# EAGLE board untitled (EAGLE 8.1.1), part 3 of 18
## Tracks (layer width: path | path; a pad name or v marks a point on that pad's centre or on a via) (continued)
S$2206 (continued)
  Bottom 0: 13.42,162.33 14.77,162.33
S$2207
  Bottom 0: 14.77,162.33 14.89,162.14
S$2208
  Bottom 0: 14.89,162.14 15.12,161.92
S$2209
  Bottom 0: 15.12,161.92 15.24,161.86
S$2210
  Bottom 0: 15.24,161.86 15.24,154.9
S$2211
  Bottom 0: 15.24,154.9 14.14,153.8
S$2212
  Bottom 0: 14.14,153.8 14.24,154.11
S$2213
  Bottom 0: 14.24,154.11 14.29,154.56
S$2214
  Bottom 0: 14.29,154.56 14.24,155.01
S$2215
  Bottom 0: 14.24,155.01 14.11,155.43
S$2216
  Bottom 0: 14.11,155.43 13.9,155.83
S$2217
  Bottom 0: 13.9,155.83 13.61,156.17
S$2218
  Bottom 0: 13.61,156.17 13.27,156.46
S$2219
  Bottom 0: 13.27,156.46 12.87,156.67
S$2220
  Bottom 0: 12.87,156.67 12.45,156.8
S$2221
  Bottom 0: 12.45,156.8 12,156.84
S$2222
  Bottom 0: 12,156.84 11.55,156.8
S$2223
  Bottom 0: 11.55,156.8 11.12,156.67
S$2224
  Bottom 0: 11.12,156.67 10.73,156.46
S$2225
  Bottom 0: 10.73,156.46 10.38,156.17
S$2226
  Bottom 0: 10.38,156.17 10.1,155.83
S$2227
  Bottom 0: 10.1,155.83 9.89,155.43
S$2228
  Bottom 0: 9.89,155.43 9.76,155.01
S$2229
  Bottom 0: 9.76,155.01 9.71,154.56
S$2230
  Bottom 0: 9.71,154.56 9.76,154.11
S$2231
  Bottom 0: 9.76,154.11 9.89,153.68
S$2232
  Bottom 0: 9.89,153.68 10.1,153.29
S$2233
  Bottom 0: 10.1,153.29 10.38,152.94
S$2234
  Bottom 0: 10.38,152.94 10.73,152.66
S$2235
  Bottom 0: 10.73,152.66 11.12,152.45
S$2236
  Bottom 0: 11.12,152.45 11.55,152.32
S$2237
  Bottom 0: 11.55,152.32 12,152.27
S$2238
  Bottom 0: 12,152.27 12.45,152.32
S$2239
  Bottom 0: 12.45,152.32 12.75,152.41
S$2240
  Bottom 0: 12.75,152.41 11.32,150.98
S$2241
  Bottom 0: 11.32,150.98 11.26,150.92
S$2242
  Bottom 0: 11.26,150.92 11.22,150.84
S$2243
  Bottom 0: 11.22,150.84 11.18,150.76
S$2244
  Bottom 0: 11.18,150.76 11.16,150.67
S$2245
  Bottom 0: 11.16,150.67 11.16,150.58
S$2246
  Bottom 0: 11.16,150.58 11.16,139.25
S$2247
  Bottom 0: 11.16,139.25 11.16,139.18
S$2248
  Bottom 0: 11.16,139.18 0.88,128.9
S$2249
  Bottom 0: 0.88,128.9 0.82,128.83
S$2250
  Bottom 0: 0.82,128.83 0.78,128.75
S$2251
  Bottom 0: 0.78,128.75 0.74,128.67
S$2252
  Bottom 0: 0.74,128.67 0.72,128.59
S$2253
  Bottom 0: 0.72,128.59 0.71,128.49
S$2254
  Bottom 0: 0.71,128.49 0.71,104.63
S$2255
  Bottom 0: 0.71,104.63 0.59,104.57
S$2256
  Bottom 0: 0.59,104.57 0.36,104.34
S$2257
  Bottom 0: 0.36,104.34 0.19,104.07
S$2258
  Bottom 0: 0.19,104.07 0.1,103.75
S$2259
  Bottom 0: 0.1,103.75 0.1,103.43
S$2260
  Bottom 0: 0.1,103.43 0.19,103.11
S$2261
  Bottom 0: 0.19,103.11 0.36,102.84
S$2262
  Bottom 0: 0.36,102.84 0.59,102.62
S$2263
  Bottom 0: 0.59,102.62 0.88,102.47
S$2264
  Bottom 0: 0.88,102.47 1.2,102.4
S$2265
  Bottom 0: 1.2,102.4 1.53,102.42
S$2266
  Bottom 0: 1.53,102.42 1.83,102.53
S$2267
  Bottom 0: 1.83,102.53 2.1,102.72
S$2268
  Bottom 0: 2.1,102.72 2.3,102.97
S$2269
  Bottom 0: 2.3,102.97 2.43,103.27
S$2270
  Bottom 0: 2.43,103.27 2.48,103.59
S$2271
  Bottom 0: 2.48,103.59 2.43,103.91
S$2272
  Bottom 0: 2.43,103.91 2.3,104.21
S$2273
  Bottom 0: 2.3,104.21 2.1,104.47
S$2274
  Bottom 0: 2.1,104.47 1.85,104.64
S$2275
  Bottom 0: 1.85,104.64 1.85,128.26
S$2276
  Bottom 0: 1.85,128.26 12.11,138.53
S$2277
  Bottom 0: 12.11,138.53 16.02,138.53
S$2278
  Bottom 0: 16.02,138.53 19.37,135.17
S$2279
  Bottom 0: 19.37,135.17 19.37,133.7
S$2280
  Bottom 0: 19.37,133.7 19.21,133.92
S$2281
  Bottom 0: 19.21,133.92 18.94,134.15
S$2282
  Bottom 0: 18.94,134.15 18.62,134.3
S$2283
  Bottom 0: 18.62,134.3 18.27,134.36
S$2284
  Bottom 0: 18.27,134.36 17.93,134.34
S$2285
  Bottom 0: 17.93,134.34 17.59,134.23
S$2286
  Bottom 0: 17.59,134.23 17.3,134.05
S$2287
  Bottom 0: 17.3,134.05 17.06,133.79
S$2288
  Bottom 0: 17.06,133.79 16.89,133.48
S$2289
  Bottom 0: 16.89,133.48 16.8,133.14
S$2290
  Bottom 0: 16.8,133.14 16.8,132.79
S$2291
  Bottom 0: 16.8,132.79 16.89,132.46
S$2292
  Bottom 0: 16.89,132.46 16.95,132.35
S$2293
  Bottom 0: 16.95,132.35 9.29,124.7
S$2294
  Bottom 0: 9.29,124.7 9.21,124.59
S$2295
  Bottom 0: 9.21,124.59 9.19,124.53
S$2296
  Bottom 0: 9.19,124.53 9.17,124.46
S$2297
  Bottom 0: 9.17,124.46 9.16,124.39
S$2298
  Bottom 0: 9.16,124.39 9.16,103.63
S$2299
  Bottom 0: 9.16,103.63 7.46,103.63
S$2300
  Bottom 0: 7.46,103.63 7.38,103.62
S$2301
  Bottom 0: 7.38,103.62 7.32,103.58
S$2302
  Bottom 0: 7.32,103.58 7.26,103.53
S$2303
  Bottom 0: 7.26,103.53 7.22,103.45
S$2304
  Bottom 0: 7.22,103.45 7.21,103.38
S$2305
  Bottom 0: 7.21,103.38 7.21,102.93
S$2306
  Bottom 0: 7.21,102.93 7.08,102.93
S$2307
  Bottom 0: 7.08,102.93 6.86,102.87
S$2308
  Bottom 0: 6.86,102.87 6.7,102.71
S$2309
  Bottom 0: 6.7,102.71 6.64,102.49
S$2310
  Bottom 0: 6.64,102.49 6.64,101.96
S$2311
  Bottom 0: 6.64,101.96 1.75,97.06
S$2312
  Bottom 0: 1.75,97.06 1.53,97.14
S$2313
  Bottom 0: 1.53,97.14 1.2,97.16
S$2314
  Bottom 0: 1.2,97.16 0.88,97.09
S$2315
  Bottom 0: 0.88,97.09 0.59,96.95
S$2316
  Bottom 0: 0.59,96.95 0.36,96.72
S$2317
  Bottom 0: 0.36,96.72 0.19,96.45
S$2318
  Bottom 0: 0.19,96.45 0.1,96.13
S$2319
  Bottom 0: 0.1,96.13 0.1,95.81
S$2320
  Bottom 0: 0.1,95.81 0.19,95.49
S$2321
  Bottom 0: 0.19,95.49 0.36,95.22
S$2322
  Bottom 0: 0.36,95.22 0.59,95
S$2323
  Bottom 0: 0.59,95 0.88,94.85
S$2324
  Bottom 0: 0.88,94.85 1.2,94.78
S$2325
  Bottom 0: 1.2,94.78 1.53,94.8
S$2326
  Bottom 0: 1.53,94.8 1.83,94.91
S$2327
  Bottom 0: 1.83,94.91 2.1,95.1
S$2328
  Bottom 0: 2.1,95.1 2.3,95.35
S$2329
  Bottom 0: 2.3,95.35 2.43,95.65
S$2330
  Bottom 0: 2.43,95.65 2.48,95.97
S$2331
  Bottom 0: 2.48,95.97 2.43,96.29
S$2332
  Bottom 0: 2.43,96.29 2.37,96.43
S$2333
  Bottom 0: 2.37,96.43 7.33,101.39
S$2334
  Bottom 0: 7.33,101.39 7.38,101.36
S$2335
  Bottom 0: 7.38,101.36 7.46,101.35
S$2336
  Bottom 0: 7.46,101.35 9.16,101.35
S$2337
  Bottom 0: 9.16,101.35 9.16,100.84
S$2338
  Bottom 0: 9.16,100.84 9.17,100.77
S$2339
  Bottom 0: 9.17,100.77 9.19,100.7
S$2340
  Bottom 0: 9.19,100.7 9.21,100.64
S$2341
  Bottom 0: 9.21,100.64 9.25,100.58
S$2342
  Bottom 0: 9.25,100.58 9.29,100.52
S$2343
  Bottom 0: 9.29,100.52 10.21,99.61
S$2344
  Bottom 0: 10.21,99.61 10.07,99.65
S$2345
  Bottom 0: 10.07,99.65 9.62,99.69
S$2346
  Bottom 0: 9.62,99.69 9.17,99.65
S$2347
  Bottom 0: 9.17,99.65 8.75,99.52
S$2348
  Bottom 0: 8.75,99.52 8.35,99.31
S$2349
  Bottom 0: 8.35,99.31 8,99.02
S$2350
  Bottom 0: 8,99.02 7.72,98.68
S$2351
  Bottom 0: 7.72,98.68 7.51,98.28
S$2352
  Bottom 0: 7.51,98.28 7.38,97.86
S$2353
  Bottom 0: 7.38,97.86 7.33,97.41
S$2354
  Bottom 0: 7.33,97.41 7.38,96.96
S$2355
  Bottom 0: 7.38,96.96 7.51,96.53
S$2356
  Bottom 0: 7.51,96.53 7.72,96.14
S$2357
  Bottom 0: 7.72,96.14 8,95.79
S$2358
  Bottom 0: 8,95.79 8.35,95.51
S$2359
  Bottom 0: 8.35,95.51 8.75,95.3
S$2360
  Bottom 0: 8.75,95.3 9.17,95.17
S$2361
  Bottom 0: 9.17,95.17 9.62,95.12
S$2362
  Bottom 0: 9.62,95.12 10.07,95.17
S$2363
  Bottom 0: 10.07,95.17 10.49,95.3
S$2364
  Bottom 0: 10.49,95.3 10.89,95.51
S$2365
  Bottom 0: 10.89,95.51 11.24,95.79
S$2366
  Bottom 0: 11.24,95.79 11.52,96.14
S$2367
  Bottom 0: 11.52,96.14 11.73,96.53
S$2368
  Bottom 0: 11.73,96.53 11.86,96.96
S$2369
  Bottom 0: 11.86,96.96 11.91,97.41
S$2370
  Bottom 0: 11.91,97.41 11.86,97.86
S$2371
  Bottom 0: 11.86,97.86 11.82,97.99
S$2372
  Bottom 0: 11.82,97.99 13.56,96.25
S$2373
  Bottom 0: 13.56,96.25 13.52,96.26
S$2374
  Bottom 0: 13.52,96.26 13.16,96.24
S$2375
  Bottom 0: 13.16,96.24 12.84,96.13
S$2376
  Bottom 0: 12.84,96.13 12.54,95.95
S$2377
  Bottom 0: 12.54,95.95 12.3,95.69
S$2378
  Bottom 0: 12.3,95.69 12.13,95.38
S$2379
  Bottom 0: 12.13,95.38 12.04,95.04
S$2380
  Bottom 0: 12.04,95.04 12.04,94.7
S$2381
  Bottom 0: 12.04,94.7 12.13,94.36
S$2382
  Bottom 0: 12.13,94.36 12.3,94.05
S$2383
  Bottom 0: 12.3,94.05 12.54,93.79
S$2384
  Bottom 0: 12.54,93.79 12.84,93.6
S$2385
  Bottom 0: 12.84,93.6 13.16,93.5
S$2386
  Bottom 0: 13.16,93.5 13.52,93.48
S$2387
  Bottom 0: 13.52,93.48 13.86,93.54
S$2388
  Bottom 0: 13.86,93.54 14.18,93.69
S$2389
  Bottom 0: 14.18,93.69 14.45,93.91
S$2390
  Bottom 0: 14.45,93.91 14.65,94.2
S$2391
  Bottom 0: 14.65,94.2 14.78,94.52
S$2392
  Bottom 0: 14.78,94.52 14.83,94.87
S$2393
  Bottom 0: 14.83,94.87 14.81,95.01
S$2394
  Bottom 0: 14.81,95.01 15.72,94.09
S$2395
  Bottom 0: 15.72,94.09 15.72,92.14
S$2396
  Bottom 0: 15.72,92.14 15.73,92.07
S$2397
  Bottom 0: 15.73,92.07 15.74,92
S$2398
  Bottom 0: 15.74,92 15.77,91.94
S$2399
  Bottom 0: 15.77,91.94 15.81,91.88
S$2400
  Bottom 0: 15.81,91.88 15.85,91.83
S$2401
  Bottom 0: 15.85,91.83 16.39,91.28
S$2402
  Bottom 0: 16.39,91.28 8.75,91.28
S$2403
  Bottom 0: 8.75,91.28 8.32,91.71
S$2404
  Bottom 0: 8.32,91.71 8.43,91.98
S$2405
  Bottom 0: 8.43,91.98 8.48,92.33
S$2406
  Bottom 0: 8.48,92.33 8.43,92.67
S$2407
  Bottom 0: 8.43,92.67 8.3,93
S$2408
  Bottom 0: 8.3,93 8.1,93.28
S$2409
  Bottom 0: 8.1,93.28 7.83,93.51
S$2410
  Bottom 0: 7.83,93.51 7.51,93.66
S$2411
  Bottom 0: 7.51,93.66 7.17,93.72
S$2412
  Bottom 0: 7.17,93.72 6.82,93.7
S$2413
  Bottom 0: 6.82,93.7 6.49,93.59
S$2414
  Bottom 0: 6.49,93.59 6.19,93.41
S$2415
  Bottom 0: 6.19,93.41 5.95,93.15
S$2416
  Bottom 0: 5.95,93.15 5.78,92.84
S$2417
  Bottom 0: 5.78,92.84 5.7,92.5
S$2418
  Bottom 0: 5.7,92.5 5.7,92.16
S$2419
  Bottom 0: 5.7,92.16 5.78,91.82
S$2420
  Bottom 0: 5.78,91.82 5.95,91.51
S$2421
  Bottom 0: 5.95,91.51 6.19,91.25
S$2422
  Bottom 0: 6.19,91.25 6.49,91.06
S$2423
  Bottom 0: 6.49,91.06 6.82,90.96
S$2424
  Bottom 0: 6.82,90.96 7.17,90.94
S$2425
  Bottom 0: 7.17,90.94 7.51,91
S$2426
  Bottom 0: 7.51,91 7.7,91.08
S$2427
  Bottom 0: 7.7,91.08 8.25,90.53
S$2428
  Bottom 0: 8.25,90.53 8.3,90.48
S$2429
  Bottom 0: 8.3,90.48 8.36,90.45
S$2430
  Bottom 0: 8.36,90.45 8.43,90.42
S$2431
  Bottom 0: 8.43,90.42 8.49,90.4
S$2432
  Bottom 0: 8.49,90.4 8.56,90.4
S$2433
  Bottom 0: 275.48,90.92 275.78,90.98
S$2434
  Bottom 0: 275.78,90.98 275.89,90.94
S$2435
  Bottom 0: 275.89,90.94 276.24,90.92
S$2436
  Bottom 0: 276.24,90.92 276.59,90.98
S$2437
  Bottom 0: 276.59,90.98 276.9,91.14
S$2438
  Bottom 0: 276.9,91.14 277.17,91.36
S$2439
  Bottom 0: 277.17,91.36 277.38,91.64
S$2440
  Bottom 0: 277.38,91.64 277.5,91.97
S$2441
  Bottom 0: 277.5,91.97 277.55,92.31
S$2442
  Bottom 0: 277.55,92.31 277.5,92.66
S$2443
  Bottom 0: 277.5,92.66 277.38,92.98
S$2444
  Bottom 0: 277.38,92.98 277.17,93.27
S$2445
  Bottom 0: 277.17,93.27 276.9,93.49
S$2446
  Bottom 0: 276.9,93.49 276.59,93.64
S$2447
  Bottom 0: 276.59,93.64 276.24,93.71
S$2448
  Bottom 0: 276.24,93.71 275.89,93.69
S$2449
  Bottom 0: 275.89,93.69 275.78,93.65
S$2450
  Bottom 0: 275.78,93.65 275.48,93.71
S$2451
  Bottom 0: 275.48,93.71 275.13,93.69
S$2452
  Bottom 0: 275.13,93.69 274.8,93.58
S$2453
  Bottom 0: 274.8,93.58 274.5,93.39
S$2454
  Bottom 0: 274.5,93.39 274.26,93.14
S$2455
  Bottom 0: 274.26,93.14 274.09,92.83
S$2456
  Bottom 0: 274.09,92.83 274.07,92.76
S$2457
  Bottom 0: 274.07,92.76 270.91,92.76
S$2458
  Bottom 0: 270.91,92.76 270.16,93.5
S$2459
  Bottom 0: 270.16,93.5 270.18,93.53
S$2460
  Bottom 0: 270.18,93.53 270.22,93.83
S$2461
  Bottom 0: 270.22,93.83 270.18,94.13
S$2462
  Bottom 0: 270.18,94.13 270.04,94.4
S$2463
  Bottom 0: 270.04,94.4 269.84,94.62
S$2464
  Bottom 0: 269.84,94.62 269.57,94.77
S$2465
  Bottom 0: 269.57,94.77 269.28,94.84
S$2466
  Bottom 0: 269.28,94.84 268.98,94.82
S$2467
  Bottom 0: 268.98,94.82 268.69,94.71
S$2468
  Bottom 0: 268.69,94.71 268.46,94.52
S$2469
  Bottom 0: 268.46,94.52 268.29,94.27
S$2470
  Bottom 0: 268.29,94.27 268.2,93.98
S$2471
  Bottom 0: 268.2,93.98 268.2,93.67
S$2472
  Bottom 0: 268.2,93.67 268.29,93.39
S$2473
  Bottom 0: 268.29,93.39 268.46,93.14
S$2474
  Bottom 0: 268.46,93.14 268.69,92.95
S$2475
  Bottom 0: 268.69,92.95 268.98,92.84
S$2476
  Bottom 0: 268.98,92.84 269.28,92.82
S$2477
  Bottom 0: 269.28,92.82 269.53,92.87
S$2478
  Bottom 0: 269.53,92.87 270.4,92
S$2479
  Bottom 0: 270.4,92 270.46,91.96
S$2480
  Bottom 0: 270.46,91.96 270.52,91.92
S$2481
  Bottom 0: 270.52,91.92 270.58,91.89
S$2482
  Bottom 0: 270.58,91.89 270.65,91.88
S$2483
  Bottom 0: 270.65,91.88 270.72,91.87
S$2484
  Bottom 0: 270.72,91.87 274.07,91.87
S$2485
  Bottom 0: 274.07,91.87 274.09,91.8
S$2486
  Bottom 0: 274.09,91.8 274.26,91.49
S$2487
  Bottom 0: 274.26,91.49 274.5,91.24
S$2488
  Bottom 0: 274.5,91.24 274.8,91.05
S$2489
  Bottom 0: 274.8,91.05 275.13,90.94
S$2490
  Bottom 0: 275.13,90.94 275.48,90.92
S$2491
  Bottom 0: 197.67,90.94 198.01,91
S$2492
  Bottom 0: 198.01,91 198.33,91.15
S$2493
  Bottom 0: 198.33,91.15 198.6,91.37
S$2494
  Bottom 0: 198.6,91.37 198.81,91.66
S$2495
  Bottom 0: 198.81,91.66 198.93,91.98
S$2496
  Bottom 0: 198.93,91.98 198.98,92.33
S$2497
  Bottom 0: 198.98,92.33 198.93,92.67
S$2498
  Bottom 0: 198.93,92.67 198.81,93
S$2499
  Bottom 0: 198.81,93 198.6,93.28
S$2500
  Bottom 0: 198.6,93.28 198.33,93.51
S$2501
  Bottom 0: 198.33,93.51 198.01,93.66
S$2502
  Bottom 0: 198.01,93.66 197.67,93.72
S$2503
  Bottom 0: 197.67,93.72 197.31,93.7
S$2504
  Bottom 0: 197.31,93.7 196.99,93.59
S$2505
  Bottom 0: 196.99,93.59 196.96,93.57
S$2506
  Bottom 0: 196.96,93.57 193.44,97.09
S$2507
  Bottom 0: 193.44,97.09 193.44,104.83
S$2508
  Bottom 0: 193.44,104.83 193.63,104.94
S$2509
  Bottom 0: 193.63,104.94 193.83,105.16
S$2510
  Bottom 0: 193.83,105.16 193.97,105.43
S$2511
  Bottom 0: 193.97,105.43 194.01,105.73
S$2512
  Bottom 0: 194.01,105.73 193.97,106.03
S$2513
  Bottom 0: 193.97,106.03 193.83,106.3
S$2514
  Bottom 0: 193.83,106.3 193.63,106.52
S$2515
  Bottom 0: 193.63,106.52 193.37,106.67
S$2516
  Bottom 0: 193.37,106.67 193.07,106.74
S$2517
  Bottom 0: 193.07,106.74 192.77,106.72
S$2518
  Bottom 0: 192.77,106.72 192.49,106.61
S$2519
  Bottom 0: 192.49,106.61 192.25,106.42
S$2520
  Bottom 0: 192.25,106.42 192.08,106.17
S$2521
  Bottom 0: 192.08,106.17 191.99,105.88
S$2522
  Bottom 0: 191.99,105.88 191.99,105.58
S$2523
  Bottom 0: 191.99,105.58 192.08,105.29
S$2524
  Bottom 0: 192.08,105.29 192.25,105.04
S$2525
  Bottom 0: 192.25,105.04 192.49,104.85
S$2526
  Bottom 0: 192.49,104.85 192.55,104.83
S$2527
  Bottom 0: 192.55,104.83 192.55,96.91
S$2528
  Bottom 0: 192.55,96.91 192.56,96.84
S$2529
  Bottom 0: 192.56,96.84 192.57,96.77
S$2530
  Bottom 0: 192.57,96.77 192.6,96.71
S$2531
  Bottom 0: 192.6,96.71 192.64,96.65
S$2532
  Bottom 0: 192.64,96.65 192.68,96.6
S$2533
  Bottom 0: 192.68,96.6 196.34,92.94
S$2534
  Bottom 0: 196.34,92.94 196.28,92.84
S$2535
  Bottom 0: 196.28,92.84 196.19,92.5
S$2536
  Bottom 0: 196.19,92.5 196.19,92.16
S$2537
  Bottom 0: 196.19,92.16 196.28,91.82
S$2538
  Bottom 0: 196.28,91.82 196.45,91.51
S$2539
  Bottom 0: 196.45,91.51 196.69,91.25
S$2540
  Bottom 0: 196.69,91.25 196.99,91.06
S$2541
  Bottom 0: 196.99,91.06 197.31,90.96
S$2542
  Bottom 0: 197.31,90.96 197.67,90.94
S$2543
  Bottom 0: 126.23,90.94 126.58,91
S$2544
  Bottom 0: 126.58,91 126.89,91.15
S$2545
  Bottom 0: 126.89,91.15 127.16,91.37
S$2546
  Bottom 0: 127.16,91.37 127.37,91.66
S$2547
  Bottom 0: 127.37,91.66 127.5,91.98
S$2548
  Bottom 0: 127.5,91.98 127.54,92.33
S$2549
  Bottom 0: 127.54,92.33 127.5,92.67
S$2550
  Bottom 0: 127.5,92.67 127.37,93
S$2551
  Bottom 0: 127.37,93 127.16,93.28
S$2552
  Bottom 0: 127.16,93.28 126.89,93.51
S$2553
  Bottom 0: 126.89,93.51 126.58,93.66
S$2554
  Bottom 0: 126.58,93.66 126.23,93.72
S$2555
  Bottom 0: 126.23,93.72 125.88,93.7
S$2556
  Bottom 0: 125.88,93.7 125.55,93.59
S$2557
  Bottom 0: 125.55,93.59 125.53,93.58
S$2558
  Bottom 0: 125.53,93.58 121.99,97.11
S$2559
  Bottom 0: 121.99,97.11 121.99,104.83
S$2560
  Bottom 0: 121.99,104.83 122.18,104.94
S$2561
  Bottom 0: 122.18,104.94 122.39,105.16
S$2562
  Bottom 0: 122.39,105.16 122.52,105.44
S$2563
  Bottom 0: 122.52,105.44 122.56,105.73
S$2564
  Bottom 0: 122.56,105.73 122.52,106.03
S$2565
  Bottom 0: 122.52,106.03 122.39,106.31
S$2566
  Bottom 0: 122.39,106.31 122.18,106.53
S$2567
  Bottom 0: 122.18,106.53 121.92,106.68
S$2568
  Bottom 0: 121.92,106.68 121.62,106.75
S$2569
  Bottom 0: 121.62,106.75 121.32,106.73
S$2570
  Bottom 0: 121.32,106.73 121.04,106.61
S$2571
  Bottom 0: 121.04,106.61 120.8,106.43
S$2572
  Bottom 0: 120.8,106.43 120.64,106.18
S$2573
  Bottom 0: 120.64,106.18 120.54,105.89
S$2574
  Bottom 0: 120.54,105.89 120.54,105.58
S$2575
  Bottom 0: 120.54,105.58 120.64,105.29
S$2576
  Bottom 0: 120.64,105.29 120.8,105.04
S$2577
  Bottom 0: 120.8,105.04 121.04,104.86
S$2578
  Bottom 0: 121.04,104.86 121.11,104.83
S$2579
  Bottom 0: 121.11,104.83 121.11,96.93
S$2580
  Bottom 0: 121.11,96.93 121.11,96.86
S$2581
  Bottom 0: 121.11,96.86 121.13,96.79
S$2582
  Bottom 0: 121.13,96.79 121.15,96.73
S$2583
  Bottom 0: 121.15,96.73 121.19,96.67
S$2584
  Bottom 0: 121.19,96.67 121.23,96.61
S$2585
  Bottom 0: 121.23,96.61 124.9,92.94
S$2586
  Bottom 0: 124.9,92.94 124.85,92.84
S$2587
  Bottom 0: 124.85,92.84 124.76,92.5
S$2588
  Bottom 0: 124.76,92.5 124.76,92.16
S$2589
  Bottom 0: 124.76,92.16 124.85,91.82
S$2590
  Bottom 0: 124.85,91.82 125.02,91.51
S$2591
  Bottom 0: 125.02,91.51 125.26,91.25
S$2592
  Bottom 0: 125.26,91.25 125.55,91.06
S$2593
  Bottom 0: 125.55,91.06 125.88,90.96
S$2594
  Bottom 0: 125.88,90.96 126.23,90.94
S$2595
  Bottom 0: 54.79,90.94 55.14,91
S$2596
  Bottom 0: 55.14,91 55.45,91.15
S$2597
  Bottom 0: 55.45,91.15 55.72,91.37
S$2598
  Bottom 0: 55.72,91.37 55.93,91.66
S$2599
  Bottom 0: 55.93,91.66 56.06,91.98
S$2600
  Bottom 0: 56.06,91.98 56.1,92.33
S$2601
  Bottom 0: 56.1,92.33 56.06,92.67
S$2602
  Bottom 0: 56.06,92.67 55.93,93
S$2603
  Bottom 0: 55.93,93 55.72,93.28
S$2604
  Bottom 0: 55.72,93.28 55.45,93.51
S$2605
  Bottom 0: 55.45,93.51 55.14,93.66
S$2606
  Bottom 0: 55.14,93.66 54.79,93.72
S$2607
  Bottom 0: 54.79,93.72 54.44,93.7
S$2608
  Bottom 0: 54.44,93.7 54.11,93.59
S$2609
  Bottom 0: 54.11,93.59 54.09,93.58
S$2610
  Bottom 0: 54.09,93.58 53.52,94.14
S$2611
  Bottom 0: 53.52,94.14 53.47,94.18
S$2612
  Bottom 0: 53.47,94.18 53.41,94.22
S$2613
  Bottom 0: 53.41,94.22 53.34,94.25
S$2614
  Bottom 0: 53.34,94.25 53.28,94.26
S$2615
  Bottom 0: 53.28,94.26 53.21,94.27
S$2616
  Bottom 0: 53.21,94.27 49.82,94.27
S$2617
  Bottom 0: 49.82,94.27 49.75,94.4
S$2618
  Bottom 0: 49.75,94.4 49.55,94.62
S$2619
  Bottom 0: 49.55,94.62 49.28,94.77
S$2620
  Bottom 0: 49.28,94.77 48.99,94.84
S$2621
  Bottom 0: 48.99,94.84 48.68,94.82
S$2622
  Bottom 0: 48.68,94.82 48.41,94.71
S$2623
  Bottom 0: 48.41,94.71 48.17,94.52
S$2624
  Bottom 0: 48.17,94.52 48,94.27
S$2625
  Bottom 0: 48,94.27 47.91,93.98
S$2626
  Bottom 0: 47.91,93.98 47.91,93.67
S$2627
  Bottom 0: 47.91,93.67 48,93.39
S$2628
  Bottom 0: 48,93.39 48.17,93.14
S$2629
  Bottom 0: 48.17,93.14 48.41,92.95
S$2630
  Bottom 0: 48.41,92.95 48.68,92.84
S$2631
  Bottom 0: 48.68,92.84 48.99,92.82
S$2632
  Bottom 0: 48.99,92.82 49.28,92.88
S$2633
  Bottom 0: 49.28,92.88 49.55,93.03
S$2634
  Bottom 0: 49.55,93.03 49.75,93.25
S$2635
  Bottom 0: 49.75,93.25 49.82,93.39
S$2636
  Bottom 0: 49.82,93.39 53.02,93.39
S$2637
  Bottom 0: 53.02,93.39 53.46,92.94
S$2638
  Bottom 0: 53.46,92.94 53.41,92.84
S$2639
  Bottom 0: 53.41,92.84 53.32,92.5
S$2640
  Bottom 0: 53.32,92.5 53.32,92.16
S$2641
  Bottom 0: 53.32,92.16 53.41,91.82
S$2642
  Bottom 0: 53.41,91.82 53.58,91.51
S$2643
  Bottom 0: 53.58,91.51 53.82,91.25
S$2644
  Bottom 0: 53.82,91.25 54.11,91.06
S$2645
  Bottom 0: 54.11,91.06 54.44,90.96
S$2646
  Bottom 0: 54.44,90.96 54.79,90.94
S$2647
  Bottom 0: 316.02,95.11 316.4,95.15
S$2648
  Bottom 0: 316.4,95.15 316.78,95.11
S$2649
  Bottom 0: 316.78,95.11 317.23,95.16
S$2650
  Bottom 0: 317.23,95.16 317.65,95.29
S$2651
  Bottom 0: 317.65,95.29 318.05,95.5
S$2652
  Bottom 0: 318.05,95.5 318.4,95.78
S$2653
  Bottom 0: 318.4,95.78 318.68,96.13
S$2654
  Bottom 0: 318.68,96.13 318.9,96.53
S$2655
  Bottom 0: 318.9,96.53 319.02,96.95
S$2656
  Bottom 0: 319.02,96.95 319.07,97.4
S$2657
  Bottom 0: 319.07,97.4 319.02,97.85
S$2658
  Bottom 0: 319.02,97.85 318.9,98.27
S$2659
  Bottom 0: 318.9,98.27 318.68,98.67
S$2660
  Bottom 0: 318.68,98.67 318.4,99.01
S$2661
  Bottom 0: 318.4,99.01 318.05,99.3
S$2662
  Bottom 0: 318.05,99.3 317.65,99.51
S$2663
  Bottom 0: 317.65,99.51 317.23,99.64
S$2664
  Bottom 0: 317.23,99.64 316.78,99.69
S$2665
  Bottom 0: 316.78,99.69 316.4,99.64
S$2666
  Bottom 0: 316.4,99.64 316.02,99.69
S$2667
  Bottom 0: 316.02,99.69 315.57,99.64
S$2668
  Bottom 0: 315.57,99.64 315.15,99.51
S$2669
  Bottom 0: 315.15,99.51 314.75,99.3
S$2670
  Bottom 0: 314.75,99.3 314.41,99.01
S$2671
  Bottom 0: 314.41,99.01 314.12,98.67
S$2672
  Bottom 0: 314.12,98.67 313.91,98.27
S$2673
  Bottom 0: 313.91,98.27 313.78,97.85
S$2674
  Bottom 0: 313.78,97.85 313.74,97.4
S$2675
  Bottom 0: 313.74,97.4 313.78,96.95
S$2676
  Bottom 0: 313.78,96.95 313.91,96.53
S$2677
  Bottom 0: 313.91,96.53 314.12,96.13
S$2678
  Bottom 0: 314.12,96.13 314.41,95.78
S$2679
  Bottom 0: 314.41,95.78 314.75,95.5
S$2680
  Bottom 0: 314.75,95.5 315.15,95.29
S$2681
  Bottom 0: 315.15,95.29 315.57,95.16
S$2682
  Bottom 0: 315.57,95.16 316.02,95.11
S$2683
  Bottom 0: 200.12,95.12 200.57,95.17
S$2684
  Bottom 0: 200.57,95.17 201,95.3
S$2685
  Bottom 0: 201,95.3 201.39,95.51
S$2686
  Bottom 0: 201.39,95.51 201.74,95.79
S$2687
  Bottom 0: 201.74,95.79 202.02,96.14
S$2688
  Bottom 0: 202.02,96.14 202.24,96.53
S$2689
  Bottom 0: 202.24,96.53 202.36,96.96
S$2690
  Bottom 0: 202.36,96.96 202.41,97.41
S$2691
  Bottom 0: 202.41,97.41 202.36,97.86
S$2692
  Bottom 0: 202.36,97.86 202.24,98.28
S$2693
  Bottom 0: 202.24,98.28 202.02,98.68
S$2694
  Bottom 0: 202.02,98.68 201.74,99.02
S$2695
  Bottom 0: 201.74,99.02 201.39,99.31
S$2696
  Bottom 0: 201.39,99.31 201,99.52
S$2697
  Bottom 0: 201,99.52 200.57,99.65
S$2698
  Bottom 0: 200.57,99.65 200.12,99.69
S$2699
  Bottom 0: 200.12,99.69 199.67,99.65
S$2700
  Bottom 0: 199.67,99.65 199.25,99.52
S$2701
  Bottom 0: 199.25,99.52 198.85,99.31
S$2702
  Bottom 0: 198.85,99.31 198.51,99.02
S$2703
  Bottom 0: 198.51,99.02 198.22,98.68
S$2704
  Bottom 0: 198.22,98.68 198.01,98.28
S$2705
  Bottom 0: 198.01,98.28 197.88,97.86
S$2706
  Bottom 0: 197.88,97.86 197.84,97.41
S$2707
  Bottom 0: 197.84,97.41 197.88,96.96
S$2708
  Bottom 0: 197.88,96.96 198.01,96.53
S$2709
  Bottom 0: 198.01,96.53 198.22,96.14
S$2710
  Bottom 0: 198.22,96.14 198.51,95.79
S$2711
  Bottom 0: 198.51,95.79 198.85,95.51
S$2712
  Bottom 0: 198.85,95.51 199.25,95.3
S$2713
  Bottom 0: 199.25,95.3 199.67,95.17
S$2714
  Bottom 0: 199.67,95.17 200.12,95.12
S$2715
  Bottom 0: 128.69,95.12 129.13,95.17
S$2716
  Bottom 0: 129.13,95.17 129.56,95.3
S$2717
  Bottom 0: 129.56,95.3 129.96,95.51
S$2718
  Bottom 0: 129.96,95.51 130.3,95.79
S$2719
  Bottom 0: 130.3,95.79 130.59,96.14
S$2720
  Bottom 0: 130.59,96.14 130.8,96.53
S$2721
  Bottom 0: 130.8,96.53 130.93,96.96
S$2722
  Bottom 0: 130.93,96.96 130.97,97.41
S$2723
  Bottom 0: 130.97,97.41 130.93,97.86
S$2724
  Bottom 0: 130.93,97.86 130.8,98.28
S$2725
  Bottom 0: 130.8,98.28 130.59,98.68
S$2726
  Bottom 0: 130.59,98.68 130.3,99.02
S$2727
  Bottom 0: 130.3,99.02 129.96,99.31
S$2728
  Bottom 0: 129.96,99.31 129.56,99.52
S$2729
  Bottom 0: 129.56,99.52 129.13,99.65
S$2730
  Bottom 0: 129.13,99.65 128.69,99.69
S$2731
  Bottom 0: 128.69,99.69 128.24,99.65
S$2732
  Bottom 0: 128.24,99.65 127.81,99.52
S$2733
  Bottom 0: 127.81,99.52 127.42,99.31
S$2734
  Bottom 0: 127.42,99.31 127.07,99.02
S$2735
  Bottom 0: 127.07,99.02 126.79,98.68
S$2736
  Bottom 0: 126.79,98.68 126.57,98.28
S$2737
  Bottom 0: 126.57,98.28 126.45,97.86
S$2738
  Bottom 0: 126.45,97.86 126.4,97.41
S$2739
  Bottom 0: 126.4,97.41 126.45,96.96
S$2740
  Bottom 0: 126.45,96.96 126.57,96.53
S$2741
  Bottom 0: 126.57,96.53 126.79,96.14
S$2742
  Bottom 0: 126.79,96.14 127.07,95.79
S$2743
  Bottom 0: 127.07,95.79 127.42,95.51
S$2744
  Bottom 0: 127.42,95.51 127.81,95.3
S$2745
  Bottom 0: 127.81,95.3 128.24,95.17
S$2746
  Bottom 0: 128.24,95.17 128.69,95.12
S$2747
  Bottom 0: 306.29,95.89 306.81,95.89
S$2748
  Bottom 0: 306.81,95.89 307.31,95.98
S$2749
  Bottom 0: 307.31,95.98 307.81,96.14
S$2750
  Bottom 0: 307.81,96.14 308.26,96.39
S$2751
  Bottom 0: 308.26,96.39 308.67,96.71
S$2752
  Bottom 0: 308.67,96.71 309.02,97.09
S$2753
  Bottom 0: 309.02,97.09 309.31,97.52
S$2754
  Bottom 0: 309.31,97.52 309.51,98
S$2755
  Bottom 0: 309.51,98 309.64,98.5
S$2756
  Bottom 0: 309.64,98.5 309.68,99.01
S$2757
  Bottom 0: 309.68,99.01 309.64,99.53
S$2758
  Bottom 0: 309.64,99.53 309.51,100.03
S$2759
  Bottom 0: 309.51,100.03 309.31,100.51
S$2760
  Bottom 0: 309.31,100.51 309.02,100.94
S$2761
  Bottom 0: 309.02,100.94 308.67,101.32
S$2762
  Bottom 0: 308.67,101.32 308.26,101.64
S$2763
  Bottom 0: 308.26,101.64 307.81,101.88
S$2764
  Bottom 0: 307.81,101.88 307.31,102.05
S$2765
  Bottom 0: 307.31,102.05 306.81,102.14
S$2766
  Bottom 0: 306.81,102.14 306.29,102.14
S$2767
  Bottom 0: 306.29,102.14 305.78,102.05
S$2768
  Bottom 0: 305.78,102.05 305.29,101.88
S$2769
  Bottom 0: 305.29,101.88 304.84,101.64
S$2770
  Bottom 0: 304.84,101.64 304.42,101.32
S$2771
  Bottom 0: 304.42,101.32 304.07,100.94
S$2772
  Bottom 0: 304.07,100.94 303.79,100.51
S$2773
  Bottom 0: 303.79,100.51 303.58,100.03
S$2774
  Bottom 0: 303.58,100.03 303.45,99.53
S$2775
  Bottom 0: 303.45,99.53 303.41,99.01
S$2776
  Bottom 0: 303.41,99.01 303.45,98.5
S$2777
  Bottom 0: 303.45,98.5 303.58,98
S$2778
  Bottom 0: 303.58,98 303.79,97.52
S$2779
  Bottom 0: 303.79,97.52 304.07,97.09
S$2780
  Bottom 0: 304.07,97.09 304.42,96.71
S$2781
  Bottom 0: 304.42,96.71 304.84,96.39
S$2782
  Bottom 0: 304.84,96.39 305.29,96.14
S$2783
  Bottom 0: 305.29,96.14 305.78,95.98
S$2784
  Bottom 0: 305.78,95.98 306.29,95.89
S$2785
  Bottom 0: 169.95,96.17 170.28,96.19
S$2786
  Bottom 0: 170.28,96.19 170.58,96.3
S$2787
  Bottom 0: 170.58,96.3 170.85,96.49
S$2788
  Bottom 0: 170.85,96.49 171.06,96.74
S$2789
  Bottom 0: 171.06,96.74 171.19,97.04
S$2790
  Bottom 0: 171.19,97.04 171.23,97.36
S$2791
  Bottom 0: 171.23,97.36 171.19,97.68
S$2792
  Bottom 0: 171.19,97.68 171.06,97.98
S$2793
  Bottom 0: 171.06,97.98 170.85,98.24
S$2794
  Bottom 0: 170.85,98.24 170.58,98.42
S$2795
  Bottom 0: 170.58,98.42 170.28,98.53
S$2796
  Bottom 0: 170.28,98.53 169.95,98.55
S$2797
  Bottom 0: 169.95,98.55 169.63,98.49
S$2798
  Bottom 0: 169.63,98.49 169.35,98.34
S$2799
  Bottom 0: 169.35,98.34 169.11,98.11
S$2800
  Bottom 0: 169.11,98.11 168.94,97.84
S$2801
  Bottom 0: 168.94,97.84 168.85,97.53
S$2802
  Bottom 0: 168.85,97.53 168.85,97.2
S$2803
  Bottom 0: 168.85,97.2 168.94,96.89
S$2804
  Bottom 0: 168.94,96.89 169.11,96.61
S$2805
  Bottom 0: 169.11,96.61 169.35,96.39
S$2806
  Bottom 0: 169.35,96.39 169.63,96.24
S$2807
  Bottom 0: 169.63,96.24 169.95,96.17
S$2808
  Bottom 0: 197.96,101.35 199.74,101.35
S$2809
  Bottom 0: 199.74,101.35 199.82,101.36
S$2810
  Bottom 0: 199.82,101.36 199.89,101.4
S$2811
  Bottom 0: 199.89,101.4 199.94,101.45
S$2812
  Bottom 0: 199.94,101.45 199.98,101.52
S$2813
  Bottom 0: 199.98,101.52 200,101.6
S$2814
  Bottom 0: 200,101.6 200,103.38
S$2815
  Bottom 0: 200,103.38 199.98,103.45
S$2816
  Bottom 0: 199.98,103.45 199.94,103.53
S$2817
  Bottom 0: 199.94,103.53 199.89,103.58
S$2818
  Bottom 0: 199.89,103.58 199.82,103.62
S$2819
  Bottom 0: 199.82,103.62 199.74,103.63
S$2820
  Bottom 0: 199.74,103.63 199.29,103.63
S$2821
  Bottom 0: 199.29,103.63 199.29,103.76
S$2822
  Bottom 0: 199.29,103.76 199.23,103.98
S$2823
  Bottom 0: 199.23,103.98 199.07,104.14
S$2824
  Bottom 0: 199.07,104.14 198.85,104.2
S$2825
  Bottom 0: 198.85,104.2 198.5,104.2
S$2826
  Bottom 0: 198.5,104.2 197.42,105.28
S$2827
  Bottom 0: 197.42,105.28 197.48,105.42
S$2828
  Bottom 0: 197.48,105.42 197.53,105.74
S$2829
  Bottom 0: 197.53,105.74 197.48,106.06
S$2830
  Bottom 0: 197.48,106.06 197.35,106.36
S$2831
  Bottom 0: 197.35,106.36 197.15,106.61
S$2832
  Bottom 0: 197.15,106.61 196.88,106.8
S$2833
  Bottom 0: 196.88,106.8 196.58,106.91
S$2834
  Bottom 0: 196.58,106.91 196.25,106.93
S$2835
  Bottom 0: 196.25,106.93 195.93,106.86
S$2836
  Bottom 0: 195.93,106.86 195.64,106.72
S$2837
  Bottom 0: 195.64,106.72 195.41,106.49
S$2838
  Bottom 0: 195.41,106.49 195.24,106.22
S$2839
  Bottom 0: 195.24,106.22 195.15,105.9
S$2840
  Bottom 0: 195.15,105.9 195.15,105.58
S$2841
  Bottom 0: 195.15,105.58 195.24,105.26
S$2842
  Bottom 0: 195.24,105.26 195.41,104.99
S$2843
  Bottom 0: 195.41,104.99 195.64,104.77
S$2844
  Bottom 0: 195.64,104.77 195.93,104.62
S$2845
  Bottom 0: 195.93,104.62 196.25,104.55
S$2846
  Bottom 0: 196.25,104.55 196.58,104.57
S$2847
  Bottom 0: 196.58,104.57 196.79,104.65
S$2848
  Bottom 0: 196.79,104.65 197.85,103.6
S$2849
  Bottom 0: 197.85,103.6 197.81,103.58
S$2850
  Bottom 0: 197.81,103.58 197.76,103.53
S$2851
  Bottom 0: 197.76,103.53 197.72,103.45
S$2852
  Bottom 0: 197.72,103.45 197.71,103.38
S$2853
  Bottom 0: 197.71,103.38 197.71,101.6
S$2854
  Bottom 0: 197.71,101.6 197.72,101.52
S$2855
  Bottom 0: 197.72,101.52 197.76,101.45
S$2856
  Bottom 0: 197.76,101.45 197.81,101.4
S$2857
  Bottom 0: 197.81,101.4 197.89,101.36
S$2858
  Bottom 0: 197.89,101.36 197.96,101.35
S$2859
  Bottom 0: 126.53,101.35 128.31,101.35
S$2860
  Bottom 0: 128.31,101.35 128.38,101.36
S$2861
  Bottom 0: 128.38,101.36 128.45,101.4
S$2862
  Bottom 0: 128.45,101.4 128.51,101.45
S$2863
  Bottom 0: 128.51,101.45 128.55,101.52
S$2864
  Bottom 0: 128.55,101.52 128.56,101.6
S$2865
  Bottom 0: 128.56,101.6 128.56,103.38
S$2866
  Bottom 0: 128.56,103.38 128.55,103.45
S$2867
  Bottom 0: 128.55,103.45 128.51,103.53
S$2868
  Bottom 0: 128.51,103.53 128.45,103.58
S$2869
  Bottom 0: 128.45,103.58 128.38,103.62
S$2870
  Bottom 0: 128.38,103.62 128.31,103.63
S$2871
  Bottom 0: 128.31,103.63 127.86,103.63
S$2872
  Bottom 0: 127.86,103.63 127.86,103.76
S$2873
  Bottom 0: 127.86,103.76 127.8,103.98
S$2874
  Bottom 0: 127.8,103.98 127.64,104.14
S$2875
  Bottom 0: 127.64,104.14 127.42,104.2
S$2876
  Bottom 0: 127.42,104.2 127.06,104.2
S$2877
  Bottom 0: 127.06,104.2 125.97,105.28
S$2878
  Bottom 0: 125.97,105.28 126.03,105.42
S$2879
  Bottom 0: 126.03,105.42 126.08,105.74
S$2880
  Bottom 0: 126.08,105.74 126.03,106.06
S$2881
  Bottom 0: 126.03,106.06 125.91,106.36
S$2882
  Bottom 0: 125.91,106.36 125.7,106.61
S$2883
  Bottom 0: 125.7,106.61 125.44,106.8
S$2884
  Bottom 0: 125.44,106.8 125.13,106.91
S$2885
  Bottom 0: 125.13,106.91 124.81,106.93
S$2886
  Bottom 0: 124.81,106.93 124.48,106.86
S$2887
  Bottom 0: 124.48,106.86 124.2,106.72
S$2888
  Bottom 0: 124.2,106.72 123.96,106.49
S$2889
  Bottom 0: 123.96,106.49 123.79,106.22
S$2890
  Bottom 0: 123.79,106.22 123.7,105.9
S$2891
  Bottom 0: 123.7,105.9 123.7,105.58
S$2892
  Bottom 0: 123.7,105.58 123.79,105.26
S$2893
  Bottom 0: 123.79,105.26 123.96,104.99
S$2894
  Bottom 0: 123.96,104.99 124.2,104.77
S$2895
  Bottom 0: 124.2,104.77 124.48,104.62
S$2896
  Bottom 0: 124.48,104.62 124.81,104.55
S$2897
  Bottom 0: 124.81,104.55 125.13,104.57
S$2898
  Bottom 0: 125.13,104.57 125.35,104.65
S$2899
  Bottom 0: 125.35,104.65 126.4,103.6
S$2900
  Bottom 0: 126.4,103.6 126.38,103.58
S$2901
  Bottom 0: 126.38,103.58 126.32,103.53
S$2902
  Bottom 0: 126.32,103.53 126.28,103.45
S$2903
  Bottom 0: 126.28,103.45 126.27,103.38
S$2904
  Bottom 0: 126.27,103.38 126.27,101.6
S$2905
  Bottom 0: 126.27,101.6 126.28,101.52
S$2906
  Bottom 0: 126.28,101.52 126.32,101.45
S$2907
  Bottom 0: 126.32,101.45 126.38,101.4
S$2908
  Bottom 0: 126.38,101.4 126.45,101.36
S$2909
  Bottom 0: 126.45,101.36 126.53,101.35
S$2910
  Bottom 0: 181,109.99 181.34,110.05
S$2911
  Bottom 0: 181.34,110.05 181.66,110.2
S$2912
  Bottom 0: 181.66,110.2 181.93,110.42
S$2913
  Bottom 0: 181.93,110.42 182.13,110.71
S$2914
  Bottom 0: 182.13,110.71 182.26,111.03
S$2915
  Bottom 0: 182.26,111.03 182.31,111.38
S$2916
  Bottom 0: 182.31,111.38 182.26,111.72
S$2917
  Bottom 0: 182.26,111.72 182.13,112.05
S$2918
  Bottom 0: 182.13,112.05 181.93,112.33
S$2919
  Bottom 0: 181.93,112.33 181.66,112.56
S$2920
  Bottom 0: 181.66,112.56 181.34,112.71
S$2921
  Bottom 0: 181.34,112.71 181,112.77
S$2922
  Bottom 0: 181,112.77 180.65,112.75
S$2923
  Bottom 0: 180.65,112.75 180.31,112.64
S$2924
  Bottom 0: 180.31,112.64 180.02,112.46
S$2925
  Bottom 0: 180.02,112.46 179.78,112.2
S$2926
  Bottom 0: 179.78,112.2 179.61,111.89
S$2927
  Bottom 0: 179.61,111.89 179.52,111.55
S$2928
  Bottom 0: 179.52,111.55 179.52,111.21
S$2929
  Bottom 0: 179.52,111.21 179.61,110.87
S$2930
  Bottom 0: 179.61,110.87 179.78,110.56
S$2931
  Bottom 0: 179.78,110.56 180.02,110.3
S$2932
  Bottom 0: 180.02,110.3 180.31,110.11
S$2933
  Bottom 0: 180.31,110.11 180.65,110.01
S$2934
  Bottom 0: 180.65,110.01 181,109.99
S$2935
  Bottom 0: 174.01,111.87 174.31,111.94
S$2936
  Bottom 0: 174.31,111.94 174.57,112.09
S$2937
  Bottom 0: 174.57,112.09 174.78,112.31
S$2938
  Bottom 0: 174.78,112.31 174.91,112.58
S$2939
  Bottom 0: 174.91,112.58 174.96,112.88
S$2940
  Bottom 0: 174.96,112.88 174.91,113.18
S$2941
  Bottom 0: 174.91,113.18 174.78,113.46
S$2942
  Bottom 0: 174.78,113.46 174.57,113.67
S$2943
  Bottom 0: 174.57,113.67 174.31,113.83
S$2944
  Bottom 0: 174.31,113.83 174.01,113.89
S$2945
  Bottom 0: 174.01,113.89 173.71,113.87
S$2946
  Bottom 0: 173.71,113.87 173.43,113.76
S$2947
  Bottom 0: 173.43,113.76 173.19,113.57
S$2948
  Bottom 0: 173.19,113.57 173.03,113.33
S$2949
  Bottom 0: 173.03,113.33 172.93,113.03
S$2950
  Bottom 0: 172.93,113.03 172.93,112.73
S$2951
  Bottom 0: 172.93,112.73 173.03,112.44
S$2952
  Bottom 0: 173.03,112.44 173.19,112.19
S$2953
  Bottom 0: 173.19,112.19 173.43,112
S$2954
  Bottom 0: 173.43,112 173.71,111.89
S$2955
  Bottom 0: 173.71,111.89 174.01,111.87
S$2956
  Bottom 0: 135.91,111.87 136.21,111.94
S$2957
  Bottom 0: 136.21,111.94 136.47,112.09
S$2958
  Bottom 0: 136.47,112.09 136.67,112.31
S$2959
  Bottom 0: 136.67,112.31 136.8,112.58
S$2960
  Bottom 0: 136.8,112.58 136.85,112.88
S$2961
  Bottom 0: 136.85,112.88 136.8,113.18
S$2962
  Bottom 0: 136.8,113.18 136.67,113.46
S$2963
  Bottom 0: 136.67,113.46 136.47,113.67
S$2964
  Bottom 0: 136.47,113.67 136.21,113.83
S$2965
  Bottom 0: 136.21,113.83 135.91,113.89
S$2966
  Bottom 0: 135.91,113.89 135.61,113.87
S$2967
  Bottom 0: 135.61,113.87 135.33,113.76
S$2968
  Bottom 0: 135.33,113.76 135.09,113.57
S$2969
  Bottom 0: 135.09,113.57 134.92,113.33
S$2970
  Bottom 0: 134.92,113.33 134.83,113.03
S$2971
  Bottom 0: 134.83,113.03 134.83,112.73
S$2972
  Bottom 0: 134.83,112.73 134.92,112.44
S$2973
  Bottom 0: 134.92,112.44 135.09,112.19
S$2974
  Bottom 0: 135.09,112.19 135.33,112
S$2975
  Bottom 0: 135.33,112 135.61,111.89
S$2976
  Bottom 0: 135.61,111.89 135.91,111.87
S$2977
  Bottom 0: 183.45,114.17 183.9,114.22
S$2978
  Bottom 0: 183.9,114.22 184.32,114.35
S$2979
  Bottom 0: 184.32,114.35 184.72,114.56
S$2980
  Bottom 0: 184.72,114.56 185.06,114.84
S$2981
  Bottom 0: 185.06,114.84 185.35,115.19
S$2982
  Bottom 0: 185.35,115.19 185.56,115.58
S$2983
  Bottom 0: 185.56,115.58 185.69,116.01
S$2984
  Bottom 0: 185.69,116.01 185.74,116.46
S$2985
  Bottom 0: 185.74,116.46 185.69,116.91
S$2986
  Bottom 0: 185.69,116.91 185.56,117.33
S$2987
  Bottom 0: 185.56,117.33 185.35,117.73
S$2988
  Bottom 0: 185.35,117.73 185.06,118.07
S$2989
  Bottom 0: 185.06,118.07 184.72,118.36
S$2990
  Bottom 0: 184.72,118.36 184.32,118.57
S$2991
  Bottom 0: 184.32,118.57 183.9,118.7
S$2992
  Bottom 0: 183.9,118.7 183.45,118.75
S$2993
  Bottom 0: 183.45,118.75 183,118.7
S$2994
  Bottom 0: 183,118.7 182.57,118.57
S$2995
  Bottom 0: 182.57,118.57 182.18,118.36
S$2996
  Bottom 0: 182.18,118.36 181.83,118.07
S$2997
  Bottom 0: 181.83,118.07 181.55,117.73
S$2998
  Bottom 0: 181.55,117.73 181.34,117.33
S$2999
  Bottom 0: 181.34,117.33 181.21,116.91
S$3000
  Bottom 0: 181.21,116.91 181.16,116.46
S$3001
  Bottom 0: 181.16,116.46 181.21,116.01
S$3002
  Bottom 0: 181.21,116.01 181.34,115.58
S$3003
  Bottom 0: 181.34,115.58 181.55,115.19
S$3004
  Bottom 0: 181.55,115.19 181.83,114.84
S$3005
  Bottom 0: 181.83,114.84 182.18,114.56
S$3006
  Bottom 0: 182.18,114.56 182.57,114.35
S$3007
  Bottom 0: 182.57,114.35 183,114.22
S$3008
  Bottom 0: 183,114.22 183.45,114.17
S$3009
  Bottom 0: 126.3,114.17 126.75,114.22
S$3010
  Bottom 0: 126.75,114.22 127.17,114.35
S$3011
  Bottom 0: 127.17,114.35 127.57,114.56
S$3012
  Bottom 0: 127.57,114.56 127.91,114.84
S$3013
  Bottom 0: 127.91,114.84 128.2,115.19
S$3014
  Bottom 0: 128.2,115.19 128.41,115.58
S$3015
  Bottom 0: 128.41,115.58 128.54,116.01
S$3016
  Bottom 0: 128.54,116.01 128.59,116.46
S$3017
  Bottom 0: 128.59,116.46 128.54,116.91
S$3018
  Bottom 0: 128.54,116.91 128.41,117.33
S$3019
  Bottom 0: 128.41,117.33 128.2,117.73
S$3020
  Bottom 0: 128.2,117.73 127.91,118.07
S$3021
  Bottom 0: 127.91,118.07 127.57,118.36
S$3022
  Bottom 0: 127.57,118.36 127.17,118.57
S$3023
  Bottom 0: 127.17,118.57 126.75,118.7
S$3024
  Bottom 0: 126.75,118.7 126.3,118.75
S$3025
  Bottom 0: 126.3,118.75 125.85,118.7
S$3026
  Bottom 0: 125.85,118.7 125.42,118.57
S$3027
  Bottom 0: 125.42,118.57 125.03,118.36
S$3028
  Bottom 0: 125.03,118.36 124.68,118.07
S$3029
  Bottom 0: 124.68,118.07 124.4,117.73
S$3030
  Bottom 0: 124.4,117.73 124.18,117.33
S$3031
  Bottom 0: 124.18,117.33 124.06,116.91
S$3032
  Bottom 0: 124.06,116.91 124.01,116.46
S$3033
  Bottom 0: 124.01,116.46 124.06,116.01
S$3034
  Bottom 0: 124.06,116.01 124.18,115.58
S$3035
  Bottom 0: 124.18,115.58 124.4,115.19
S$3036
  Bottom 0: 124.4,115.19 124.68,114.84
S$3037
  Bottom 0: 124.68,114.84 125.03,114.56
S$3038
  Bottom 0: 125.03,114.56 125.42,114.35
S$3039
  Bottom 0: 125.42,114.35 125.85,114.22
S$3040
  Bottom 0: 125.85,114.22 126.3,114.17
S$3041
  Bottom 0: 9.3,125.98 9.62,126
S$3042
  Bottom 0: 9.62,126 9.93,126.11
S$3043
  Bottom 0: 9.93,126.11 10.19,126.29
S$3044
  Bottom 0: 10.19,126.29 10.4,126.55
S$3045
  Bottom 0: 10.4,126.55 10.53,126.85
S$3046
  Bottom 0: 10.53,126.85 10.57,127.17
S$3047
  Bottom 0: 10.57,127.17 10.53,127.49
S$3048
  Bottom 0: 10.53,127.49 10.4,127.79
S$3049
  Bottom 0: 10.4,127.79 10.19,128.04
S$3050
  Bottom 0: 10.19,128.04 9.93,128.23
S$3051
  Bottom 0: 9.93,128.23 9.62,128.34
S$3052
  Bottom 0: 9.62,128.34 9.3,128.36
S$3053
  Bottom 0: 9.3,128.36 8.98,128.29
S$3054
  Bottom 0: 8.98,128.29 8.69,128.14
S$3055
  Bottom 0: 8.69,128.14 8.46,127.92
S$3056
  Bottom 0: 8.46,127.92 8.29,127.64
S$3057
  Bottom 0: 8.29,127.64 8.2,127.33
S$3058
  Bottom 0: 8.2,127.33 8.2,127
S$3059
  Bottom 0: 8.2,127 8.29,126.69
S$3060
  Bottom 0: 8.29,126.69 8.46,126.42
S$3061
  Bottom 0: 8.46,126.42 8.69,126.19
S$3062
  Bottom 0: 8.69,126.19 8.98,126.05
S$3063
  Bottom 0: 8.98,126.05 9.3,125.98
S$3064
  Bottom 0: 11.93,129.04 12.27,129.1
S$3065
  Bottom 0: 12.27,129.1 12.59,129.25
S$3066
  Bottom 0: 12.59,129.25 12.86,129.47
S$3067
  Bottom 0: 12.86,129.47 13.07,129.76
S$3068
  Bottom 0: 13.07,129.76 13.19,130.08
S$3069
  Bottom 0: 13.19,130.08 13.24,130.43
S$3070
  Bottom 0: 13.24,130.43 13.19,130.77
S$3071
  Bottom 0: 13.19,130.77 13.07,131.1
S$3072
  Bottom 0: 13.07,131.1 12.86,131.38
S$3073
  Bottom 0: 12.86,131.38 12.59,131.61
S$3074
  Bottom 0: 12.59,131.61 12.27,131.76
S$3075
  Bottom 0: 12.27,131.76 11.93,131.82
S$3076
  Bottom 0: 11.93,131.82 11.57,131.8
S$3077
  Bottom 0: 11.57,131.8 11.24,131.69
S$3078
  Bottom 0: 11.24,131.69 10.95,131.51
S$3079
  Bottom 0: 10.95,131.51 10.71,131.25
S$3080
  Bottom 0: 10.71,131.25 10.54,130.94
S$3081
  Bottom 0: 10.54,130.94 10.46,130.6
S$3082
  Bottom 0: 10.46,130.6 10.46,130.25
S$3083
  Bottom 0: 10.46,130.25 10.54,129.92
S$3084
  Bottom 0: 10.54,129.92 10.71,129.61
S$3085
  Bottom 0: 10.71,129.61 10.95,129.35
S$3086
  Bottom 0: 10.95,129.35 11.24,129.16
S$3087
  Bottom 0: 11.24,129.16 11.57,129.06
S$3088
  Bottom 0: 11.57,129.06 11.93,129.04
S$3089
  Bottom 0: 14.38,133.22 14.83,133.27
S$3090
  Bottom 0: 14.83,133.27 15.26,133.4
S$3091
  Bottom 0: 15.26,133.4 15.65,133.61
S$3092
  Bottom 0: 15.65,133.61 16,133.89
S$3093
  Bottom 0: 16,133.89 16.28,134.24
S$3094
  Bottom 0: 16.28,134.24 16.5,134.63
S$3095
  Bottom 0: 16.5,134.63 16.62,135.06
S$3096
  Bottom 0: 16.62,135.06 16.67,135.51
S$3097
  Bottom 0: 16.67,135.51 16.62,135.96
S$3098
  Bottom 0: 16.62,135.96 16.5,136.38
S$3099
  Bottom 0: 16.5,136.38 16.28,136.78
S$3100
  Bottom 0: 16.28,136.78 16,137.12
S$3101
  Bottom 0: 16,137.12 15.65,137.41
S$3102
  Bottom 0: 15.65,137.41 15.26,137.62
S$3103
  Bottom 0: 15.26,137.62 14.83,137.75
S$3104
  Bottom 0: 14.83,137.75 14.38,137.79
S$3105
  Bottom 0: 14.38,137.79 13.93,137.75
S$3106
  Bottom 0: 13.93,137.75 13.51,137.62
S$3107
  Bottom 0: 13.51,137.62 13.11,137.41
S$3108
  Bottom 0: 13.11,137.41 12.76,137.12
S$3109
  Bottom 0: 12.76,137.12 12.48,136.78
S$3110
  Bottom 0: 12.48,136.78 12.27,136.38
S$3111
  Bottom 0: 12.27,136.38 12.14,135.96
S$3112
  Bottom 0: 12.14,135.96 12.1,135.51
S$3113
  Bottom 0: 12.1,135.51 12.14,135.06
S$3114
  Bottom 0: 12.14,135.06 12.27,134.63
S$3115
  Bottom 0: 12.27,134.63 12.48,134.24
S$3116
  Bottom 0: 12.48,134.24 12.76,133.89
S$3117
  Bottom 0: 12.76,133.89 13.11,133.61
S$3118
  Bottom 0: 13.11,133.61 13.51,133.4
S$3119
  Bottom 0: 13.51,133.4 13.93,133.27
S$3120
  Bottom 0: 13.93,133.27 14.38,133.22
S$3121
  Bottom 0: 9.3,142.65 9.62,142.67
S$3122
  Bottom 0: 9.62,142.67 9.93,142.78
S$3123
  Bottom 0: 9.93,142.78 10.19,142.97
S$3124
  Bottom 0: 10.19,142.97 10.4,143.22
S$3125
  Bottom 0: 10.4,143.22 10.53,143.52
S$3126
  Bottom 0: 10.53,143.52 10.57,143.84
S$3127
  Bottom 0: 10.57,143.84 10.53,144.16
S$3128
  Bottom 0: 10.53,144.16 10.4,144.46
S$3129
  Bottom 0: 10.4,144.46 10.19,144.71
S$3130
  Bottom 0: 10.19,144.71 9.93,144.9
S$3131
  Bottom 0: 9.93,144.9 9.62,145.01
S$3132
  Bottom 0: 9.62,145.01 9.3,145.03
S$3133
  Bottom 0: 9.3,145.03 8.98,144.96
S$3134
  Bottom 0: 8.98,144.96 8.69,144.82
S$3135
  Bottom 0: 8.69,144.82 8.46,144.59
S$3136
  Bottom 0: 8.46,144.59 8.29,144.32
S$3137
  Bottom 0: 8.29,144.32 8.2,144
S$3138
  Bottom 0: 8.2,144 8.2,143.68
S$3139
  Bottom 0: 8.2,143.68 8.29,143.36
S$3140
  Bottom 0: 8.29,143.36 8.46,143.09
S$3141
  Bottom 0: 8.46,143.09 8.69,142.87
S$3142
  Bottom 0: 8.69,142.87 8.98,142.72
S$3143
  Bottom 0: 8.98,142.72 9.3,142.65
S$3144
  Bottom 0: 9.54,148.09 9.89,148.15
S$3145
  Bottom 0: 9.89,148.15 10.21,148.3
S$3146
  Bottom 0: 10.21,148.3 10.47,148.52
S$3147
  Bottom 0: 10.47,148.52 10.68,148.81
S$3148
  Bottom 0: 10.68,148.81 10.81,149.13
S$3149
  Bottom 0: 10.81,149.13 10.86,149.48
S$3150
  Bottom 0: 10.86,149.48 10.81,149.82
S$3151
  Bottom 0: 10.81,149.82 10.68,150.15
S$3152
  Bottom 0: 10.68,150.15 10.47,150.43
S$3153
  Bottom 0: 10.47,150.43 10.21,150.66
S$3154
  Bottom 0: 10.21,150.66 9.89,150.81
S$3155
  Bottom 0: 9.89,150.81 9.54,150.87
S$3156
  Bottom 0: 9.54,150.87 9.19,150.85
S$3157
  Bottom 0: 9.19,150.85 8.86,150.74
S$3158
  Bottom 0: 8.86,150.74 8.57,150.56
S$3159
  Bottom 0: 8.57,150.56 8.33,150.3
S$3160
  Bottom 0: 8.33,150.3 8.16,149.99
S$3161
  Bottom 0: 8.16,149.99 8.07,149.65
S$3162
  Bottom 0: 8.07,149.65 8.07,149.3
S$3163
  Bottom 0: 8.07,149.3 8.16,148.97
S$3164
  Bottom 0: 8.16,148.97 8.33,148.66
S$3165
  Bottom 0: 8.33,148.66 8.57,148.4
S$3166
  Bottom 0: 8.57,148.4 8.86,148.21
S$3167
  Bottom 0: 8.86,148.21 9.19,148.11
S$3168
  Bottom 0: 9.19,148.11 9.54,148.09
S$3169
  Bottom 0: 9.84,158.5 11.62,158.5
S$3170
  Bottom 0: 11.62,158.5 11.69,158.51
S$3171
  Bottom 0: 11.69,158.51 11.76,158.55
S$3172
  Bottom 0: 11.76,158.55 11.82,158.6
S$3173
  Bottom 0: 11.82,158.6 11.86,158.67
S$3174
  Bottom 0: 11.86,158.67 11.87,158.75
S$3175
  Bottom 0: 11.87,158.75 11.87,160.53
S$3176
  Bottom 0: 11.87,160.53 11.86,160.6
S$3177
  Bottom 0: 11.86,160.6 11.82,160.68
S$3178
  Bottom 0: 11.82,160.68 11.76,160.73
S$3179
  Bottom 0: 11.76,160.73 11.69,160.77
S$3180
  Bottom 0: 11.69,160.77 11.62,160.78
S$3181
  Bottom 0: 11.62,160.78 11.17,160.78
S$3182
  Bottom 0: 11.17,160.78 11.17,160.91
S$3183
  Bottom 0: 11.17,160.91 11.11,161.13
S$3184
  Bottom 0: 11.11,161.13 10.95,161.29
S$3185
  Bottom 0: 10.95,161.29 10.73,161.35
S$3186
  Bottom 0: 10.73,161.35 10.37,161.35
S$3187
  Bottom 0: 10.37,161.35 9.28,162.44
S$3188
  Bottom 0: 9.28,162.44 9.34,162.57
S$3189
  Bottom 0: 9.34,162.57 9.38,162.89
S$3190
  Bottom 0: 9.38,162.89 9.34,163.22
S$3191
  Bottom 0: 9.34,163.22 9.21,163.51
S$3192
  Bottom 0: 9.21,163.51 9,163.77
S$3193
  Bottom 0: 9,163.77 8.74,163.96
S$3194
  Bottom 0: 8.74,163.96 8.44,164.06
S$3195
  Bottom 0: 8.44,164.06 8.11,164.08
S$3196
  Bottom 0: 8.11,164.08 7.79,164.02
S$3197
  Bottom 0: 7.79,164.02 7.5,163.87
S$3198
  Bottom 0: 7.5,163.87 7.27,163.65
S$3199
  Bottom 0: 7.27,163.65 7.1,163.37
S$3200
  Bottom 0: 7.1,163.37 7.01,163.06
S$3201
  Bottom 0: 7.01,163.06 7.01,162.73
S$3202
  Bottom 0: 7.01,162.73 7.1,162.42
S$3203
  Bottom 0: 7.1,162.42 7.27,162.14
S$3204
  Bottom 0: 7.27,162.14 7.5,161.92
S$3205
  Bottom 0: 7.5,161.92 7.79,161.77
S$3206
  Bottom 0: 7.79,161.77 8.11,161.71
S$3207
  Bottom 0: 8.11,161.71 8.44,161.73
S$3208
  Bottom 0: 8.44,161.73 8.65,161.8
S$3209
  Bottom 0: 8.65,161.8 9.71,160.75
S$3210
  Bottom 0: 9.71,160.75 9.69,160.73
S$3211
  Bottom 0: 9.69,160.73 9.64,160.68
S$3212
  Bottom 0: 9.64,160.68 9.59,160.6
S$3213
  Bottom 0: 9.59,160.6 9.59,160.53
S$3214
  Bottom 0: 9.59,160.53 9.59,158.75
S$3215
  Bottom 0: 9.59,158.75 9.59,158.67
S$3216
  Bottom 0: 9.59,158.67 9.64,158.6
S$3217
  Bottom 0: 9.64,158.6 9.69,158.55
S$3218
  Bottom 0: 9.69,158.55 9.76,158.51
S$3219
  Bottom 0: 9.76,158.51 9.84,158.5
S$3220
  Bottom 0: 39.55,161.71 39.87,161.73
S$3221
  Bottom 0: 39.87,161.73 40.17,161.83
S$3222
  Bottom 0: 40.17,161.83 40.44,162.02
S$3223
  Bottom 0: 40.44,162.02 40.65,162.28
S$3224
  Bottom 0: 40.65,162.28 40.67,162.33
S$3225
  Bottom 0: 40.67,162.33 46.77,162.33
S$3226
  Bottom 0: 46.77,162.33 46.86,162.33
S$3227
  Bottom 0: 46.86,162.33 46.95,162.35
S$3228
  Bottom 0: 46.95,162.35 47.03,162.38
S$3229
  Bottom 0: 47.03,162.38 47.11,162.43
S$3230
  Bottom 0: 47.11,162.43 47.18,162.49
S$3231
  Bottom 0: 47.18,162.49 48.82,164.13
S$3232
  Bottom 0: 48.82,164.13 49.07,164.08
S$3233
  Bottom 0: 49.07,164.08 49.4,164.1
S$3234
  Bottom 0: 49.4,164.1 49.7,164.21
S$3235
  Bottom 0: 49.7,164.21 49.97,164.39
S$3236
  Bottom 0: 49.97,164.39 50.17,164.65
S$3237
  Bottom 0: 50.17,164.65 50.2,164.7
S$3238
  Bottom 0: 50.2,164.7 56.07,164.7
S$3239
  Bottom 0: 56.07,164.7 57.54,163.24
S$3240
  Bottom 0: 57.54,163.24 57.49,163.06
S$3241
  Bottom 0: 57.49,163.06 57.49,162.74
S$3242
  Bottom 0: 57.49,162.74 57.58,162.42
S$3243
  Bottom 0: 57.58,162.42 57.76,162.15
S$3244
  Bottom 0: 57.76,162.15 57.99,161.93
S$3245
  Bottom 0: 57.99,161.93 58.28,161.78
S$3246
  Bottom 0: 58.28,161.78 58.6,161.71
S$3247
  Bottom 0: 58.6,161.71 58.92,161.73
S$3248
  Bottom 0: 58.92,161.73 59.23,161.84
S$3249
  Bottom 0: 59.23,161.84 59.49,162.03
S$3250
  Bottom 0: 59.49,162.03 59.7,162.28
S$3251
  Bottom 0: 59.7,162.28 59.83,162.58
S$3252
  Bottom 0: 59.83,162.58 59.87,162.9
S$3253
  Bottom 0: 59.87,162.9 59.83,163.22
S$3254
  Bottom 0: 59.83,163.22 59.7,163.52
S$3255
  Bottom 0: 59.7,163.52 59.49,163.77
S$3256
  Bottom 0: 59.49,163.77 59.23,163.96
S$3257
  Bottom 0: 59.23,163.96 58.92,164.07
S$3258
  Bottom 0: 58.92,164.07 58.6,164.09
S$3259
  Bottom 0: 58.6,164.09 58.34,164.04
S$3260
  Bottom 0: 58.34,164.04 56.71,165.67
S$3261
  Bottom 0: 56.71,165.67 56.64,165.73
S$3262
  Bottom 0: 56.64,165.73 56.57,165.78
S$3263
  Bottom 0: 56.57,165.78 56.48,165.81
S$3264
  Bottom 0: 56.48,165.81 56.39,165.83
S$3265
  Bottom 0: 56.39,165.83 56.3,165.84
S$3266
  Bottom 0: 56.3,165.84 50.2,165.84
S$3267
  Bottom 0: 50.2,165.84 50.17,165.89
S$3268
  Bottom 0: 50.17,165.89 49.97,166.14
S$3269
  Bottom 0: 49.97,166.14 49.7,166.33
S$3270
  Bottom 0: 49.7,166.33 49.4,166.44
S$3271
  Bottom 0: 49.4,166.44 49.07,166.46
S$3272
  Bottom 0: 49.07,166.46 48.75,166.39
S$3273
  Bottom 0: 48.75,166.39 48.46,166.24
S$3274
  Bottom 0: 48.46,166.24 48.23,166.02
S$3275
  Bottom 0: 48.23,166.02 48.06,165.75
S$3276
  Bottom 0: 48.06,165.75 47.97,165.43
S$3277
  Bottom 0: 47.97,165.43 47.97,165.1
S$3278
  Bottom 0: 47.97,165.1 48.01,164.94
S$3279
  Bottom 0: 48.01,164.94 46.54,163.46
S$3280
  Bottom 0: 46.54,163.46 40.67,163.46
S$3281
  Bottom 0: 40.67,163.46 40.65,163.51
S$3282
  Bottom 0: 40.65,163.51 40.44,163.77
S$3283
  Bottom 0: 40.44,163.77 40.17,163.96
S$3284
  Bottom 0: 40.17,163.96 39.87,164.06
S$3285
  Bottom 0: 39.87,164.06 39.55,164.08
S$3286
  Bottom 0: 39.55,164.08 39.29,164.03
S$3287
  Bottom 0: 39.29,164.03 37.65,165.67
S$3288
  Bottom 0: 37.65,165.67 37.59,165.74
S$3289
  Bottom 0: 37.59,165.74 37.51,165.78
S$3290
  Bottom 0: 37.51,165.78 37.43,165.81
S$3291
  Bottom 0: 37.43,165.81 37.34,165.84
S$3292
  Bottom 0: 37.34,165.84 37.25,165.84
S$3293
  Bottom 0: 37.25,165.84 31.14,165.84
S$3294
  Bottom 0: 31.14,165.84 31.12,165.89
S$3295
  Bottom 0: 31.12,165.89 30.91,166.15
S$3296
  Bottom 0: 30.91,166.15 30.65,166.33
S$3297
  Bottom 0: 30.65,166.33 30.34,166.44
S$3298
  Bottom 0: 30.34,166.44 30.02,166.46
S$3299
  Bottom 0: 30.02,166.46 29.7,166.4
S$3300
  Bottom 0: 29.7,166.4 29.41,166.25
S$3301
  Bottom 0: 29.41,166.25 29.17,166.03
S$3302
  Bottom 0: 29.17,166.03 29,165.75
S$3303
  Bottom 0: 29,165.75 28.91,165.43
S$3304
  Bottom 0: 28.91,165.43 28.91,165.11
S$3305
  Bottom 0: 28.91,165.11 29,164.79
S$3306
  Bottom 0: 29,164.79 29.17,164.52
S$3307
  Bottom 0: 29.17,164.52 29.41,164.3
S$3308
  Bottom 0: 29.41,164.3 29.7,164.15
S$3309
  Bottom 0: 29.7,164.15 30.02,164.08
S$3310
  Bottom 0: 30.02,164.08 30.34,164.1
S$3311
  Bottom 0: 30.34,164.1 30.65,164.21
S$3312
  Bottom 0: 30.65,164.21 30.91,164.4
S$3313
  Bottom 0: 30.91,164.4 31.12,164.65
S$3314
  Bottom 0: 31.12,164.65 31.14,164.7
S$3315
  Bottom 0: 31.14,164.7 37.02,164.7
S$3316
  Bottom 0: 37.02,164.7 38.49,163.23
S$3317
  Bottom 0: 38.49,163.23 38.45,163.06
S$3318
  Bottom 0: 38.45,163.06 38.45,162.73
S$3319
  Bottom 0: 38.45,162.73 38.53,162.42
S$3320
  Bottom 0: 38.53,162.42 38.7,162.14
S$3321
  Bottom 0: 38.7,162.14 38.94,161.92
S$3322
  Bottom 0: 38.94,161.92 39.23,161.77
S$3323
  Bottom 0: 39.23,161.77 39.55,161.71
S$3324
  Bottom 0: 231.97,164.08 232.29,164.1
S$3325
  Bottom 0: 232.29,164.1 232.6,164.21
S$3326
  Bottom 0: 232.6,164.21 232.86,164.39
S$3327
  Bottom 0: 232.86,164.39 233.07,164.65
S$3328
